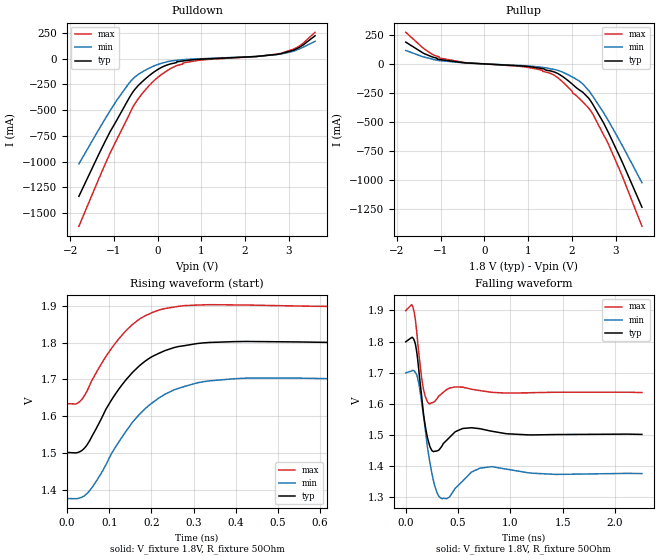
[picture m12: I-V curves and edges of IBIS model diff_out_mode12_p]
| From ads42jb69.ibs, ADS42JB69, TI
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|   diff_out_mode12 Model
[Model]   diff_out_mode12_p
Model_type   Output
Polarity   Non-Inverting
Vmeas = 1.659
Vref = 1.8
Cref = 0.5pF
Rref = 50
|   typ   min   max
|   (nom PVT)   (fast PVT)   (slow PVT)
C_comp   2.611e-12   2.311e-12   2.731e-12
[Model Spec]
Vmeas   1.659   1.56   1.757
| Where nom  PVT is Nominal Process, 1.8V, 25C
|   Fast PVT is Strong Process,  1.9V, -40C
|   Slow PVT is Weak Process,   1.7V, 120C
[Voltage Range]   1.8   1.7   1.9
[Temperature Range]   25   120   -40
[Pullup Reference]   1.8   1.7   1.9
[Pulldown Reference]   0   0   0
[Power Clamp Reference]   1.8   1.7   1.9
[GND Clamp Reference]   0   0   0
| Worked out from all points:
|   slope of the pulldown table from 0 to 0.27 V, typ, clamps not added: 5.18 ohm
|   slope of the pullup table from 0 to 0.27 V, typ, clamps not added: 49.4 ohm
|   falling waveform, V_fixture 1.8V, R_fixture 50Ohm: 20-80 % time 57.2ps typ, 77.2ps min, 49.7ps max; typ from 1.8 V to 1.5 V
|   rising waveform, V_fixture 1.8V, R_fixture 50Ohm: 20-80 % time 107ps typ, 120ps min, 97ps max; typ from 1.5 V to 1.8 V
[Pulldown]
|   Voltage   I(typ)   I(min)   I(max)
-1.8V     -1.336A    -1.021A    -1.627A
-1.089V   -710.8mA   -506.3mA   -918.4mA
-618.5mV  -358.3mA   -219.8mA   -514.9mA
-536.4mV  -306.2mA   -183.8mA   -448.2mA
-373.1mV  -231.6mA   -133.7mA   -350.4mA
-1.8mV    -106.4mA   -57.01mA   -183.2mA
316.5mV   -48.43mA   -21.37mA   -91.53mA
621mV     -19.52mA   -8.364mA   -38.77mA
1.082V    -2.543mA   1.491mA    -9.459mA
2.819V    48.74mA    46.01mA    51.78mA
3.237V    109.3mA    94.39mA    121.5mA
3.6V      222.8mA    168.4mA    256.6mA
[Pullup]
|   Voltage   I(typ)   I(min)   I(max)
-1.8V     187.8mA    116mA      272.7mA
-1.368V   87.07mA    57.51mA    126.7mA
-1.034V   37.99mA    28.94mA    51.33mA
-450mV    9.292mA    7.813mA    11.7mA
1.005V    -22.9mA    -18.07mA   -31.06mA
1.325V    -40.4mA    -30.03mA   -54.96mA
1.694V    -86.71mA   -57.49mA   -124.8mA
2.154V    -220.6mA   -144.8mA   -292.8mA
2.474V    -346.5mA   -276.7mA   -430.6mA
2.831V    -590.1mA   -488.5mA   -689.3mA
3.168V    -862.6mA   -716.5mA   -984.7mA
3.6V      -1.235A    -1.024A    -1.4A
[Ramp]
R_load = 50
|   typ   min   max
dV/dt_r   0.0865636/6.1839e-11   0.11304/7.7745e-11   0.0700682/5.38318e-11
dV/dt_f   0.178438/5.71777e-11   0.193852/7.66144e-11   0.157877/4.94486e-11
[Falling Waveform]
V_fixture = 1.8V
V_fixture_min = 1.7V
V_fixture_max = 1.9V
R_fixture = 50Ohm
|   Time   V(typ)   V(min)   V(max)
0s        1.799V     1.699V     1.899V
56ps      1.813V     1.706V     1.918V
90ps      1.795V     1.702V     1.875V
150ps     1.63V      1.609V     1.688V
206ps     1.494V     1.464V     1.607V
276ps     1.448V     1.338V     1.608V
344ps     1.463V     1.296V     1.633V
544ps     1.521V     1.352V     1.654V
814ps     1.513V     1.398V     1.637V
2.258ns   1.502V     1.376V     1.636V
[Rising Waveform]
V_fixture = 1.8V
V_fixture_min = 1.7V
V_fixture_max = 1.9V
R_fixture = 50Ohm
|   Time   V(typ)   V(min)   V(max)
0s        1.501V     1.376V     1.635V
26ps      1.501V     1.376V     1.636V
52ps      1.53V      1.395V     1.68V
80ps      1.59V      1.442V     1.74V
108ps     1.649V     1.503V     1.789V
170ps     1.735V     1.603V     1.863V
232ps     1.778V     1.659V     1.893V
308ps     1.797V     1.69V      1.902V
428ps     1.803V     1.703V     1.902V
1.414ns   1.799V     1.698V     1.899V
